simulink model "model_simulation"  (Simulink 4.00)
settings: Solver=VariableStepDiscrete  StartTime=0.0  StopTime=ts  RelTol=1e-3
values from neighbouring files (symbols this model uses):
  A = [0.9944 -0.1203 -0.4302    [model.m]
  Ao1 = A - K1*c1    [model.m]
  Ao2 = A - K2*c2    [model.m]
  Ao3 = A - K3*c3    [model.m]
  B = [0.4252 -0.0082 0.1813]'    [model.m]
  Bo1 = [B K1]    [model.m]
  Bo2 = [B K2]    [model.m]
  Bo3 = [B K3]    [model.m]
  C = eye(3)    [model.m]
  Co1 = c1    [model.m]
  Co2 = c2    [model.m]
  Co3 = c3    [model.m]
  D = zeros(3,1)    [model.m]
  Do1 = zeros(1,2)    [model.m]
  Do2 = zeros(1,2)    [model.m]
  Do3 = zeros(1,2)    [model.m]
  tf1 = ts/2    (= 25)    [model.m]
  tf2 = ts/2    (= 25)    [model.m]
  tf3 = ts/2    (= 25)    [model.m]
  x0 = [0.05 0.15 0.2]    [model.m]

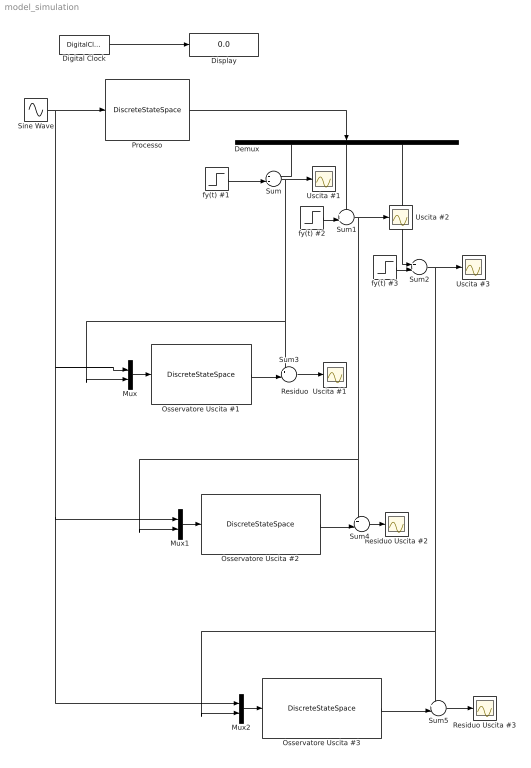
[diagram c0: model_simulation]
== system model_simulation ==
  Demux : Demux  Orientation=down  Outputs=3  BusSelectionMode=off
  Digital Clock : DigitalClock  SampleTime=0.1
  Display : Display
  Mux : Mux  Inputs=2
  Mux1 : Mux  Inputs=2
  Mux2 : Mux  Inputs=2
  Osservatore Uscita #1 : DiscreteStateSpace  A=Ao1  B=Bo1  C=Co1  D=Do1  X0=0  SampleTime=0.1  Realization=auto
  Osservatore Uscita #2 : DiscreteStateSpace  A=Ao2  B=Bo2  C=Co2  D=Do2  X0=0  SampleTime=0.1  Realization=auto
  Osservatore Uscita #3 : DiscreteStateSpace  A=Ao3  B=Bo3  C=Co3  D=Do3  X0=0  SampleTime=0.1  Realization=auto
  Processo : DiscreteStateSpace  A=A  B=B  C=C  D=D  X0=x0  SampleTime=0.1  Realization=auto
  Residuo Uscita #2 : Scope
  Residuo Uscita #3 : Scope
  Residuo  Uscita #1 : Scope
  Sine Wave : Sin  SineType=Time-based  Amplitude=1  Bias=0  Frequency=1  Phase=0  Samples=10  SampleTime=0.01
  Sum : Sum  Inputs=++|  SaturateOnIntegerOverflow=on
  Sum1 : Sum  Inputs=++|  SaturateOnIntegerOverflow=on
  Sum2 : Sum  Inputs=++|  SaturateOnIntegerOverflow=on
  Sum3 : Sum  Inputs=+-|  SaturateOnIntegerOverflow=on
  Sum4 : Sum  Inputs=+-|  SaturateOnIntegerOverflow=on
  Sum5 : Sum  Inputs=+-|  SaturateOnIntegerOverflow=on
  Uscita #1 : Scope
  Uscita #2 : Scope
  Uscita #3 : Scope
  fy(t) #1 : Step  Time=tf1  Before=0  After=1  SampleTime=0.1
  fy(t) #2 : Step  Time=tf2  Before=0  After=1  SampleTime=0.1
  fy(t) #3 : Step  Time=tf3  Before=0  After=1  SampleTime=0.1
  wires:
  Sine Wave/1 -> Processo/1, Mux/1, Mux1/1, Mux2/1
  Processo/1 -> Demux/1
  Osservatore Uscita #1/1 -> Sum3/2
  Mux/1 -> Osservatore Uscita #1/1
  Demux/1 -> Sum/1
  Demux/2 -> Sum1/1
  Demux/3 -> Sum2/1
  Digital Clock/1 -> Display/1
  Sum/1 -> Uscita #1/1, Mux/2, Sum3/1
  Sum1/1 -> Uscita #2/1, Sum4/1, Mux1/2
  Sum2/1 -> Uscita #3/1, Mux2/2, Sum5/1
  fy(t) #1/1 -> Sum/2
  Sum3/1 -> Residuo  Uscita #1/1
  Osservatore Uscita #2/1 -> Sum4/2
  Mux1/1 -> Osservatore Uscita #2/1
  Sum4/1 -> Residuo Uscita #2/1
  fy(t) #2/1 -> Sum1/2
  fy(t) #3/1 -> Sum2/2
  Osservatore Uscita #3/1 -> Sum5/2
  Mux2/1 -> Osservatore Uscita #3/1
  Sum5/1 -> Residuo Uscita #3/1
